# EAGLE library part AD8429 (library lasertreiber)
AD8429 Datasheet
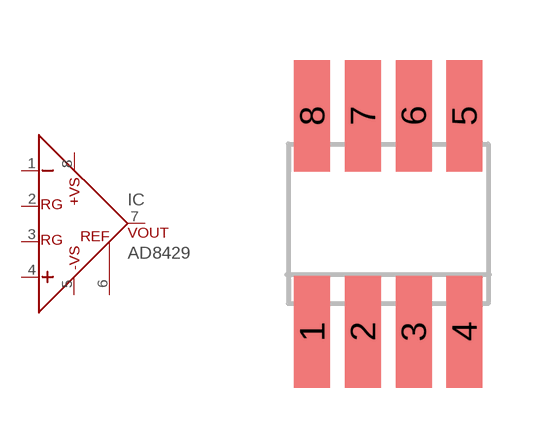
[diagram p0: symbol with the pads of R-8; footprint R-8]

Designator prefix IC

## AD8429  [R-8]
1  -IN  in
2  RG  pas
3  RG  pas
4  +IN  in
5  -VIN  pwr
6  REF  pas
7  VOUT  out
8  +VIN  pwr

## Footprint R-8 (pad centres in mm)
smd 0.9 x 2.8: 1 -1.905,-2.7; 2 -0.635,-2.7; 3 0.635,-2.7; 4 1.905,-2.7; 5 1.905,2.7; 6 0.635,2.7; 7 -0.635,2.7; 8 -1.905,2.7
